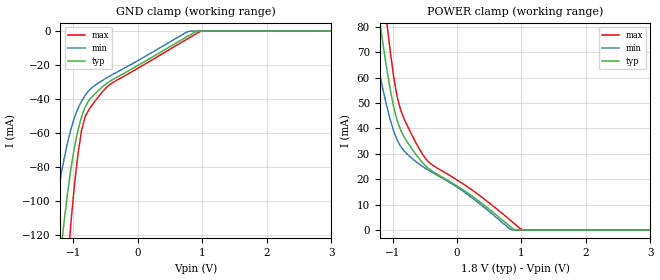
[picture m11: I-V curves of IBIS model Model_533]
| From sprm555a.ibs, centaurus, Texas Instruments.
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| Model based on original model for BCSHTLTCSCDDVPBFZ_SSGFV
|   Sub model DIFF_VREF_FULLTERM_9MA_10PER_1P8
[model]   Model_533
|[Description]  [1.8V-INPUT-FULLTERM:9MA-X, IND, 10%]
|   FULLTERM, 0.88 * RExt = 1.125 * Iout (I[2:0] = "100"), 9mA
|   nominal with Rext = 50R,Industrial temperature range (-40C to
|   125C, 25C nominal),10% power supply tolerance
|[Input Load]   FULLTERM:9MA
|[Output Drive]
|Voltage   1.8V
|Mode   INPUT
Model_type   Input
Polarity   Non-Inverting
Vinl =  0.775
Vinh =  1.025
C_comp   1.851324p   1.663768p   1.973575p
[Model Spec]
Vinl   0.775   0.685   0.865
Vinh   1.025   0.935   1.115
[Temperature Range]   25   125   -40
[Voltage Range]   1.8   1.62   1.98
[POWER_clamp]
-1.8V     207.1mA    145.5mA    278.4mA
-1.364V   114.3mA    82.67mA    150.5mA
-1.309V   103.4mA    75.4mA     135.7mA
-1.2V     82.51mA    61.48mA    107.8mA
-1.145V   72.74mA    54.96mA    94.58mA
-1.091V   63.64mA    48.9mA     82.07mA
-981.8mV  48.41mA    38.91mA    60.25mA
-872.7mV  39.22mA    32.88mA    47.15mA
-545.5mV  26.81mA    25.21mA    30.25mA
818.2mV   1.492mA    381.5uA    4.024mA
1.036V    0A         0A         0A
3.6V      0A         0A         0A
[GND_clamp]
-1.8V     -367.8mA   -226.9mA   -591.6mA
-1.364V   -192.7mA   -122.2mA   -303.8mA
-1.145V   -113.1mA   -75.68mA   -169.2mA
-1.091V   -95.74mA   -65.93mA   -139.1mA
-1.036V   -80.57mA   -57.56mA   -112.4mA
-927.3mV  -58.19mA   -45.46mA   -72.08mA
-872.7mV  -50.53mA   -41.27mA   -58.66mA
-763.6mV  -41.17mA   -35.22mA   -46.58mA
-436.4mV  -29.61mA   -26.52mA   -31.57mA
763.6mV   -3.28mA    -460.8uA   -4.735mA
981.8mV   0A         0A         0A
3.6V      0A         0A         0A
